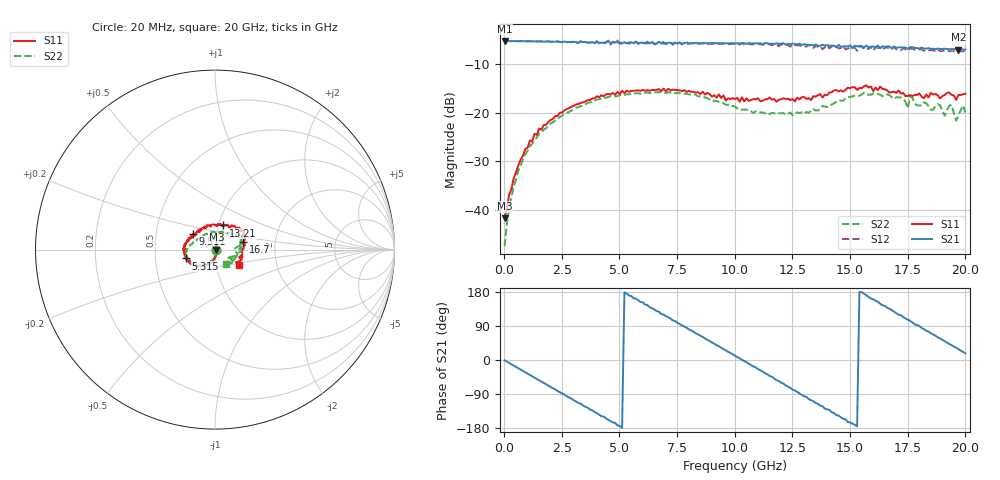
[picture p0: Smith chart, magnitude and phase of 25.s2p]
!Agilent Technologies,N5230A,US43500223,A.07.50.48
!Agilent N5230A: A.07.50.48
!Date: Thursday, October 08, 2015 12:17:50
!Correction: S11(Full 2 Port(1,2))
!S21(Full 2 Port(1,2))
!S12(Full 2 Port(1,2))
!S22(Full 2 Port(1,2))
!S2P File: Measurements: S11, S21, S12, S22:
# Hz S  RI  R 50
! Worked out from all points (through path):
!   201 points, 20 MHz to 20 GHz, reference 50 ohm
!   highest |S21| = -5.13 dB at 20 MHz (marker M1); lowest = -6.9 dB at 19.7 GHz (marker M2)
!   group delay of S21, straight-line fit = 97.4 ps
!   lowest |S11| = -41.8 dB at 20 MHz (marker M3), VSWR 1.02, Z = 50.8 + j0.0173 ohm
!   |S11| at or under -10 dB: start of sweep to end of sweep
!   |S22| runs from -47.6 to -15.7 dB; largest |S21 - S12| = 0.061
!   S11 on the Smith chart (normalised r, x): 20 MHz: 1.02, +0.00; 5.315 GHz: 0.72, -0.07; 9.511 GHz: 0.77, +0.14; 13.21 GHz: 1.05, +0.29; 16.7 GHz: 1.36, +0.12; 20 GHz: 1.28, -0.23
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2e7  0.00808 0.00017  0.5538 -0.00719  0.5529 -0.00763  0.00406 -0.001
4.196e8  0.00855 -0.0194  0.5329 -0.142  0.5321 -0.1433  0.00504 -0.0167
9.191e8  0.00353 -0.0422  0.4641 -0.2955  0.4621 -0.2971  -0.00208 -0.0373
2.3177e9  -0.044 -0.0816  0.0759 -0.5419  0.0696 -0.5416  -0.0403 -0.0763
3.4166e9  -0.0887 -0.0921  -0.2677 -0.4651  -0.2833 -0.4546  -0.0798 -0.0874
4.5155e9  -0.1345 -0.0803  -0.5082 -0.2097  -0.5218 -0.2023  -0.1208 -0.0803
5.3147e9  -0.1623 -0.0493  -0.5216 0.0413  -0.5229 0.0624  -0.1416 -0.0653
6.7133e9  -0.1755 -0.00806  -0.3301 0.4284  -0.3144 0.4332  -0.1597 -0.0298
7.9121e9  -0.1608 0.0332  0.0438 0.5315  0.069 0.5113  -0.1574 0.000211
9.5105e9  -0.124 0.087  0.4574 0.2535  0.4623 0.2303  -0.1173 0.0454
1.001e10  -0.1001 0.0964  0.5117 0.1008  0.508 0.0788  -0.1021 0.0553
1.18082e10  -0.0234 0.1281  0.3132 -0.4201  0.2834 -0.4185  -0.0296 0.0932
1.32068e10  0.0446 0.1346  -0.1156 -0.4904  -0.1433 -0.4861  0.0296 0.0953
1.34066e10  0.0501 0.1397  -0.1604 -0.4715  -0.1757 -0.4333  0.042 0.1009
1.54046e10  0.1463 0.1067  -0.4854 0.00664  -0.4954 -0.00845  0.1313 0.0722
1.67033e10  0.1559 0.0435  -0.347 0.3411  -0.3028 0.3356  0.1481 0.0349
1.81019e10  0.1433 -0.0325  0.0442 0.4707  0.0608 0.4472  0.1183 -0.0138
1.89011e10  0.1219 -0.0703  0.2504 0.382  0.2612 0.345  0.1014 -0.0635
1.91009e10  0.138 -0.0653  0.2977 0.3516  0.2997 0.3212  0.0835 -0.0412
1.94006e10  0.1289 -0.0832  0.3503 0.2889  0.355 0.2562  0.0941 -0.0756
1.97003e10  0.1304 -0.0807  0.3968 0.214  0.3974 0.1867  0.0826 -0.0421
2e10  0.1321 -0.0863  0.4303 0.1354  0.4225 0.1057  0.0622 -0.079
